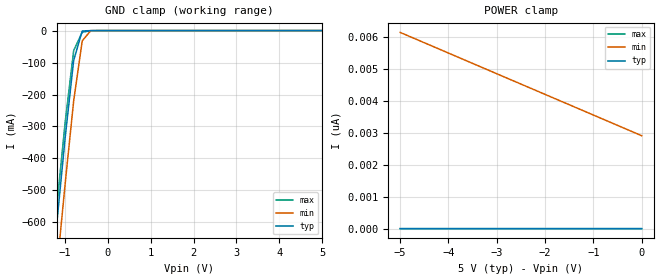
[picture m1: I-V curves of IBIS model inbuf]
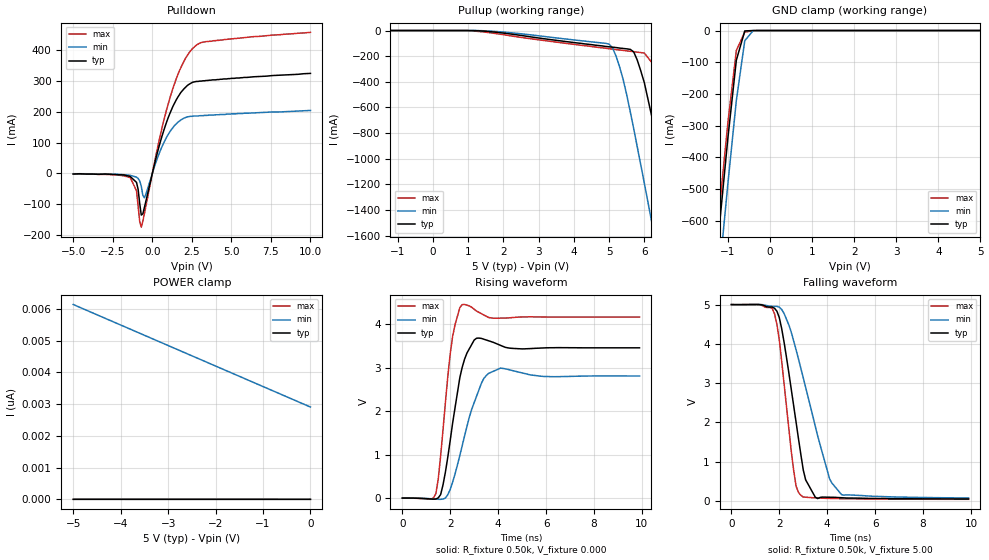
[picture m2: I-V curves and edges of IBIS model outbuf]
| IBIS file 41574k.ibs created by s2ibis2 version 1.0
| North Carolina State University Electronics Research Laboratory  1995
[IBIS ver]   2.1
[File name]   41574k.ibs
[File Rev]   0.1
[Date]   Friday, July 11, 1997
[Source]   IDT
[Notes]   1. Temp typ=25C, min=100C, max=0C 2. Ramp rates based on 500
   ohm load
[Copyright]   Copyright 1997, Integrated Device Technology, Inc.
|   Component IDT54/74FCT574T/AT/CT
[Component]   IDT54/74FCT574T/AT/CT
[Manufacturer]   Integrated Device Technology Inc.
[Package]
| Following package parameters are for D20-1(CDIP), P20-1(DPIP) packages
|[Package]
|| variable   typ   min   max
|R_pkg   40.00m   30.00m   50.00m
|L_pkg   7.00nH   4.00nH   10.00nH
|C_pkg   0.60pF   0.50pF   0.70pF
| Following package parameters are for SO20-6(EIAJ), SO20-2(SOIC) packages
|[Package]
|| variable   typ   min   max
|R_pkg   25.00m   20.00m   30.00m
|L_pkg   3.50nH   2.10nH   6.50nH
|C_pkg   0.40pF   0.35pF   0.60pF
| Following package parameters are for SO20-8(QSOP), SO20-7(SSOP) packages
| variable   typ   min   max
R_pkg   20.00m   15.00m   25.00m
L_pkg   3.00nH   2.00nH   4.00nH
C_pkg   0.30pF   0.26pF   0.34pF
[Pin]  signal_name   model_name   R_pin   L_pin   C_pin
1   OEB   inbuf
2   D0   inbuf
3   D1   inbuf
4   D2   inbuf
5   D3   inbuf
6   D4   inbuf
7   D5   inbuf
8   D6   inbuf
9   D7   inbuf
10   GND   GND
11   CP   inbuf
12   Q7   outbuf
13   Q6   outbuf
14   Q5   outbuf
15   Q4   outbuf
16   Q3   outbuf
17   Q2   outbuf
18   Q1   outbuf
19   Q0   outbuf
20   VCC   POWER
| Models and submodels in the file (2): inbuf (Input), outbuf (I/O)
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| in   IN1   dummy_model
| oe   OE1   dummy_model
|   Model inbuf
[Model]   inbuf
Model_type   Input
Vinl =  0.800V
Vinh =  2.000V
C_comp   3.00pF   NA   NA
[Temperature Range]   25.00   100.00   0.000
[Voltage Range]   5.00V   4.50V   5.50V
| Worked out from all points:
|   GND clamp passes 1 mA (typ) near -0.55 V on its own axis
[GND_clamp]
| voltage   I(typ)   I(min)   I(max)
-5V       -6.185A    -6.347A    -6.076A
-1.4V     -895mA     -1.042A    -839mA
-1.2V     -612mA     -758mA     -559mA
-1V       -337mA     -481mA     -289mA
-800mV    -93.47mA   -220mA     -62.86mA
-600mV    -1.292mA   -32.12mA   -4.905mA
-400mV    -309nA     -162uA     -673uA
5V        467fA      3.231nA    197fA
[POWER_clamp]
| voltage   I(typ)   I(min)   I(max)
-5V       993fA      6.14nA     489fA
-4.5V     943fA      5.816nA    465fA
-4.2V     910fA      5.623nA    450fA
0V        467fA      2.908nA    227fA
|   Model outbuf
[Model]   outbuf
Model_type   I/O
Polarity   Non-Inverting
Enable   Active-High
Vinl =  0.800V
Vinh =  2.000V
C_comp   3.00pF   NA   NA
[Temperature Range]   25.00   100.00   0.000
[Voltage Range]   5.00V   4.50V   5.50V
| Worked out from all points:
|   slope of the pulldown table from 0 to 0.75 V, typ, clamps not added: 5.24 ohm
|   GND clamp passes 1 mA (typ) near -0.55 V on its own axis
|   rising waveform, R_fixture 0.50k, V_fixture 0.000: 20-80 % time 573ps typ, 830ps min, 429ps max; typ from 0 V to 3.46 V
|   falling waveform, R_fixture 0.50k, V_fixture 5.00: 20-80 % time 728ps typ, 1.25ns min, 530ps max; typ from 5 V to 0.048 V
[Pulldown]
| voltage   I(typ)   I(min)   I(max)
-5V       -2mA       -1mA       -2mA
-1.4V     -9.8mA     -6mA       -13.3mA
-1V       -29mA      -12.1mA    -56.2mA
-800mV    -96.13mA   -24.2mA    -155mA
-700mV    -135mA     -41.5mA    -174mA
-500mV    -110mA     -79.11mA   -130mA
300mV     63.4mA     46.63mA    75.9mA
900mV     166mA      117mA      206mA
1.7V      254mA      169mA      331mA
2.5V      294mA      185mA      402mA
3.4V      301mA      188mA      427mA
10V       324mA      204mA      457mA
[Pullup]
| voltage   I(typ)   I(min)   I(max)
-5V       0A         0A         0A
1V        -8.847nA   2.262nA    -1.224mA
5V        -127mA     -106mA     -142mA
5.2V      -133mA     -202mA     -149mA
5.4V      -140mA     -382mA     -155mA
5.7V      -167mA     -768mA     -165mA
6V        -407mA     -1.191A    -176mA
6.4V      -905mA     -1.769A    -315mA
6.8V      -1.477A    -2.353A    -719mA
7.2V      -2.058A    -2.941A    -1.274A
7.6V      -2.644A    -3.531A    -1.847A
10V       -6.186A    -7.091A    -5.345A
[GND_clamp]
| voltage   I(typ)   I(min)   I(max)
-5V       -6.185A    -6.347A    -6.076A
-1.4V     -895mA     -1.042A    -839mA
-1.2V     -612mA     -758mA     -559mA
-1V       -337mA     -481mA     -289mA
-800mV    -93.47mA   -220mA     -62.86mA
-600mV    -1.292mA   -32.12mA   -4.905mA
-400mV    -309nA     -162uA     -673uA
5V        466fA      3.231nA    198fA
[POWER_clamp]
| voltage   I(typ)   I(min)   I(max)
-5V       989fA      6.14nA     490fA
-4.5V     939fA      5.816nA    467fA
-4.2V     910fA      5.623nA    450fA
0V        465fA      2.908nA    226fA
[Ramp]
| variable   typ   min   max
dV/dt_r   2.07/0.57n   1.68/0.83n   2.50/0.43n
dV/dt_f   2.97/0.73n   2.66/1.16n   3.27/0.57n
R_load = 0.50k
[Rising Waveform]
R_fixture = 0.50k
V_fixture = 0.000
| time   V(typ)   V(min)   V(max)
0s        0V         0V         0V
1.4ns     -21.29mV   -24.12mV   101mV
1.5ns     4.917mV    -28.22mV   437mV
1.7ns     308mV      -21.9mV    1.58V
2.1ns     1.725V     365mV      3.72V
2.5ns     3.009V     1.206V     4.449V
3ns       3.634V     2.196V     4.341V
3.3ns     3.671V     2.639V     4.24V
4.1ns     3.511V     2.989V     4.138V
9.9ns     3.455V     2.807V     4.162V
[Falling Waveform]
R_fixture = 0.50k
V_fixture = 5.00
| time   V(typ)   V(min)   V(max)
0s        5V         5V         5V
1.8ns     4.906V     4.956V     4.766V
2.1ns     4.386V     4.877V     3.553V
2.6ns     2.422V     4.072V     774mV
2.9ns     1.179V     3.374V     143mV
3.1ns     535mV      2.887V     93.33mV
3.5ns     96.1mV     1.907V     76.58mV
4.1ns     92.8mV     560mV      62.66mV
4.6ns     80.03mV    158mV      56.01mV
9.9ns     48.12mV    74.23mV    39.36mV
